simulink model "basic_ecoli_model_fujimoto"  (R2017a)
settings: Solver=ode45  StartTime=6.69  StopTime=11.57  MaxStep=0.001  RelTol=1e-6  AbsTol=1e-6  EnableMultiTasking=on
undefined symbols (not defined in the file or in its folder): F, K1, Ks, Mmax, S0, So, V, X0

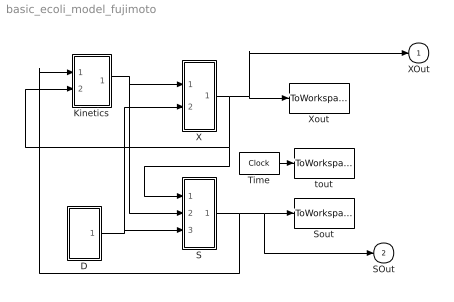
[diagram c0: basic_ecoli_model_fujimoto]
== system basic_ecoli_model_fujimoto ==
  D : Subsystem
  Kinetics : Subsystem
  S : Subsystem
  Sout : ToWorkspace  VariableName=Sout  SampleTime=-1
  Time : Clock
  X : Subsystem
  Xout : ToWorkspace  VariableName=Xout  SampleTime=-1
  tout : ToWorkspace  VariableName=tout  SampleTime=-1
  XOut : Outport
  SOut : Outport  Port=2
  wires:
  X/1(XOut) -> Xout/1, XOut/1, Kinetics/2(X), S/1(X)
  S/1(Sout) -> Kinetics/1(S), Sout/1, SOut/1
  Time/1 -> tout/1
  Kinetics/1(mu) -> X/1(mu), S/2(mu)
  D/1(out_1) -> S/3(F/V), X/2(F/V)

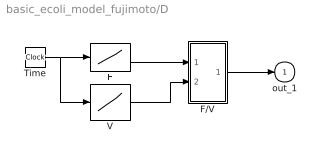
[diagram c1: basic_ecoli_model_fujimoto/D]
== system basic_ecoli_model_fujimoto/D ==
  F : Lookup  InputValues=t  Table=F
  F/V : Subsystem
  Time : Clock
  V : Lookup  InputValues=t  Table=V
  out_1 : Outport
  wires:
  F/V/1(out_1) -> out_1/1
  F/1 -> F/V/1(F)
  V/1 -> F/V/2(V)
  Time/1 -> F/1, V/1

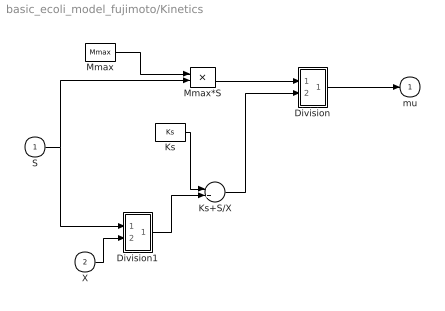
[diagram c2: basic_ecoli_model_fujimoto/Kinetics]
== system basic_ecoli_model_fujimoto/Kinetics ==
  S : Inport
  X : Inport  Port=2
  Division : Subsystem
  Division1 : Subsystem
  Ks : Constant  Value=Ks
  Ks+S/X : Sum
  Mmax : Constant  Value=Mmax
  Mmax*S : Product
  mu : Outport
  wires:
  Division/1(out_1) -> mu/1
  Mmax/1 -> Mmax*S/1
  Mmax*S/1 -> Division/1(Mmax*S)
  Ks+S/X/1 -> Division/2(Ks+S)
  S/1 -> Division1/1(Mmax*S), Mmax*S/2
  Ks/1 -> Ks+S/X/1
  X/1 -> Division1/2(Ks+S)
  Division1/1(out_1) -> Ks+S/X/2

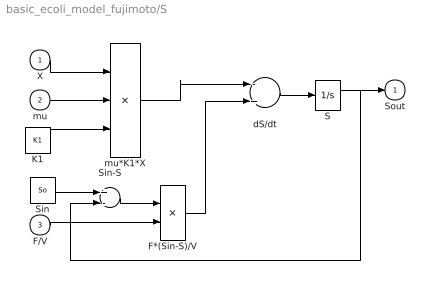
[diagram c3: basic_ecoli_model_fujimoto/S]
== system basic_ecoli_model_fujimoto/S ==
  X : Inport
  mu : Inport  Port=2
  F/V : Inport  Port=3
  F*(Sin-S)/V : Product
  K1 : Constant  Value=K1
  S : Integrator  InitialCondition=S0  UpperSaturationLimit=1000  LowerSaturationLimit=0
  Sin : Constant  Value=So
  Sin-S : Sum  Inputs=+-
  dS/dt : Sum  Inputs=-+
  mu*K1*X : Product  Inputs=3
  Sout : Outport
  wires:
  S/1 -> Sout/1, Sin-S/2
  Sin-S/1 -> F*(Sin-S)/V/1
  Sin/1 -> Sin-S/1
  X/1 -> mu*K1*X/1
  F/V/1 -> F*(Sin-S)/V/2
  mu*K1*X/1 -> dS/dt/1
  F*(Sin-S)/V/1 -> dS/dt/2
  dS/dt/1 -> S/1
  mu/1 -> mu*K1*X/2
  K1/1 -> mu*K1*X/3

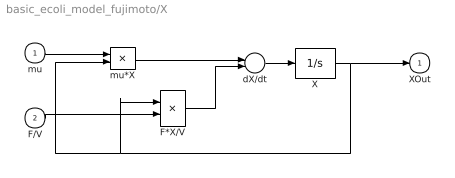
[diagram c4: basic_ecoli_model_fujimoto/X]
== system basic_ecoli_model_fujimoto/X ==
  mu : Inport
  F/V : Inport  Port=2
  F*X/V : Product
  X : Integrator  InitialCondition=X0  UpperSaturationLimit=1000  LowerSaturationLimit=0
  dX/dt : Sum  Inputs=+-
  mu*X : Product
  XOut : Outport
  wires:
  F*X/V/1 -> dX/dt/2
  dX/dt/1 -> X/1
  mu*X/1 -> dX/dt/1
  mu/1 -> mu*X/1
  X/1 -> XOut/1, mu*X/2, F*X/V/1
  F/V/1 -> F*X/V/2

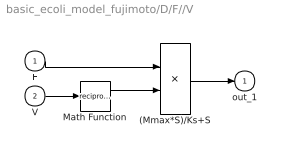
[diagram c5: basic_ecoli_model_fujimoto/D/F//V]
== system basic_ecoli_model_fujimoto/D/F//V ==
  F : Inport
  V : Inport  Port=2
  (Mmax*S)/Ks+S : Product
  Math Function : Math  Operator=reciprocal
  out_1 : Outport
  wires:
  F/1 -> (Mmax*S)/Ks+S/1
  V/1 -> Math Function/1
  Math Function/1 -> (Mmax*S)/Ks+S/2
  (Mmax*S)/Ks+S/1 -> out_1/1

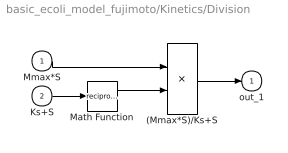
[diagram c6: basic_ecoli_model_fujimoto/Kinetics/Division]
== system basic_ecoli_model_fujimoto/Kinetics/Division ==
  Mmax*S : Inport
  Ks+S : Inport  Port=2
  (Mmax*S)/Ks+S : Product
  Math Function : Math  Operator=reciprocal
  out_1 : Outport
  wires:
  Mmax*S/1 -> (Mmax*S)/Ks+S/1
  Ks+S/1 -> Math Function/1
  Math Function/1 -> (Mmax*S)/Ks+S/2
  (Mmax*S)/Ks+S/1 -> out_1/1

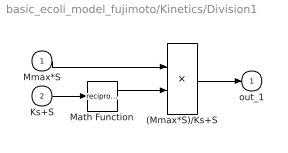
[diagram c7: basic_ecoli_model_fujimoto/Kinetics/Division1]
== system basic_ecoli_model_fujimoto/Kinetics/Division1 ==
  Mmax*S : Inport
  Ks+S : Inport  Port=2
  (Mmax*S)/Ks+S : Product
  Math Function : Math  Operator=reciprocal
  out_1 : Outport
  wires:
  Mmax*S/1 -> (Mmax*S)/Ks+S/1
  Ks+S/1 -> Math Function/1
  Math Function/1 -> (Mmax*S)/Ks+S/2
  (Mmax*S)/Ks+S/1 -> out_1/1
